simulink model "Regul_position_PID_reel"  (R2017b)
settings: Solver=ode5  StartTime=0.0  StopTime=inf  FixedStep=0.005  RelTol=1e-3  AbsTol=1e-6
undefined symbols (not defined in the file or in its folder): RTDAC4PCIBaseAddress

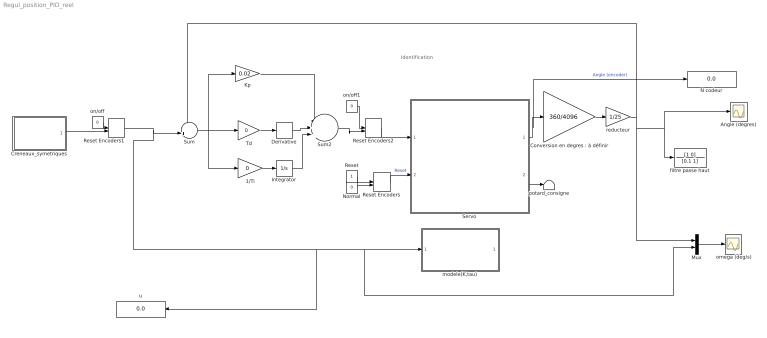
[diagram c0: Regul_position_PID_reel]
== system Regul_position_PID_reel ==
  note: Identification
  " omega (deg/s)" : Scope
  1/Ti : Gain  Gain=0
  Angle (degres) : Scope
  "Conversion en degres : à définir" : Gain  Gain=360/4096
  Creneaux_symetriques : Subsystem
  Derivative : Derivative
  Integrator : Integrator
  Kp : Gain  Gain=0.02
  Mux : Mux  Inputs=2
  N codeur : Display
  Normal : Constant  Value=0
  Reset : Constant
  Reset Encoders : ManualSwitch  CurrentSetting=0
  Reset Encoders1 : ManualSwitch  CurrentSetting=0
  Reset Encoders2 : ManualSwitch  CurrentSetting=0
  Servo : Subsystem  mask{BaseAddress=RTDAC4PCIBaseAddress(-1,-1), T0=0.005}
      mask prompts: BaseAddress "Base Address:"; T0 "Sampling Period:"
  Sum : Sum  Inputs=-+|
  Sum2 : Sum  Inputs=|+||+|+||
  Td : Gain  Gain=0
  filtre passe haut : TransferFcn  Numerator=[1 0]  Denominator=[0.1 1]
  modele(K,tau) : Subsystem
  on/off : Constant  Value=0
  on/off1 : Constant  Value=0
  potard_consigne : Terminator
  reducteur : Gain  Gain=1/25
  u : Display
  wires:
  Reset Encoders/1 -> Servo/2(Reset Encoder)  "Reset"
  Normal/1 -> Reset Encoders/2
  Reset/1 -> Reset Encoders/1
  Servo/2(Set-up) -> potard_consigne/1
  Servo/1(Codeur_angulaire) -> N codeur/1, "Conversion en degres : à définir"/1  "Angle (encoder)"
  "Conversion en degres : à définir"/1 -> reducteur/1
  Mux/1 -> " omega (deg/s)"/1
  on/off/1 -> Reset Encoders1/1
  Creneaux_symetriques/1(u) -> Reset Encoders1/2
  Reset Encoders1/1 -> Sum/2, Mux/2, modele(K,tau)/1(u), u/1
  Td/1 -> Derivative/1
  Integrator/1 -> Sum2/3
  Derivative/1 -> Sum2/2
  Kp/1 -> Sum2/1
  1/Ti/1 -> Integrator/1
  Sum/1 -> 1/Ti/1, Kp/1, Td/1
  reducteur/1 -> Mux/1, Angle (degres)/1, filtre passe haut/1, Sum/1
  Sum2/1 -> Reset Encoders2/2
  Reset Encoders2/1 -> Servo/1(PWM Control)
  on/off1/1 -> Reset Encoders2/1

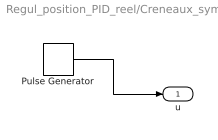
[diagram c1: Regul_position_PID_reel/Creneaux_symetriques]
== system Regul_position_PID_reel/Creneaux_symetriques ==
  Pulse Generator : DiscretePulseGenerator  PulseType=Time based  Amplitude=20  Period=0.005*floor(15/0.005)  PulseWidth=50  PhaseDelay=0.005*floor(0*15/0.005/4)
  u : Outport
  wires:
  Pulse Generator/1 -> u/1

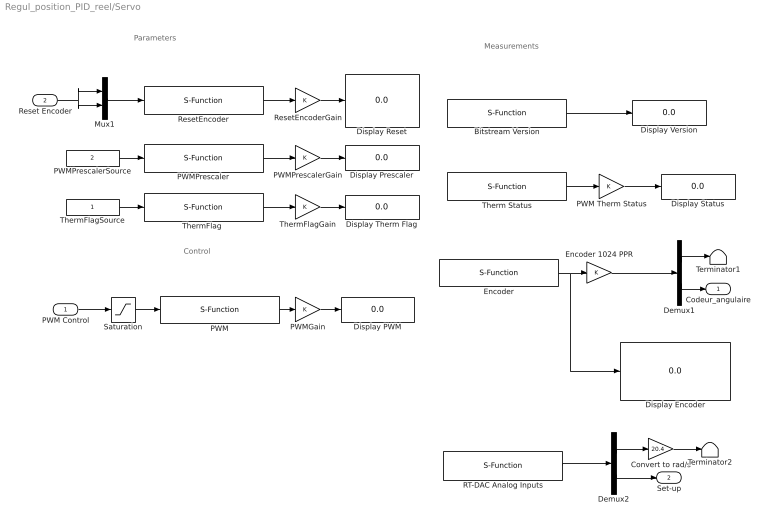
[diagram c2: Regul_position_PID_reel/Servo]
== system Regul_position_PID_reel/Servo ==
  note: Parameters
  note: Control
  note: Measurements
  PWM Control : Inport
  Reset Encoder : Inport  Port=2
  Bitstream Version : S-Function  FunctionName=Servo_BitstreamVersion  Parameters=BaseAddress, T0  SFunctionDeploymentMode=off  EnableBusSupport=off
  Convert to rad/s : Gain  Gain=20.4
  Demux1 : Demux  Outputs=2
  Demux2 : Demux  Outputs=2
  Display Encoder : Display
  Display PWM : Display
  Display Prescaler : Display
  Display Reset : Display
  Display Status : Display
  Display Therm Flag : Display
  Display Version : Display
  Encoder : S-Function  FunctionName=Servo_Encoder  Parameters=BaseAddress, T0  SFunctionDeploymentMode=off  EnableBusSupport=off
  Encoder 1024 PPR : Gain
  Mux1 : Mux  Inputs=2
  PWM : S-Function  FunctionName=Servo_PWM  Parameters=BaseAddress, T0  SFunctionDeploymentMode=off  EnableBusSupport=off
  PWM Therm Status : Gain
  PWMGain : Gain
  PWMPrescaler : S-Function  FunctionName=Servo_PWMPrescaler  Parameters=BaseAddress, T0  SFunctionDeploymentMode=off  EnableBusSupport=off
  PWMPrescalerGain : Gain
  PWMPrescalerSource : Constant  Value=2
  RT-DAC Analog Inputs : S-Function  FunctionName=servo_analoginputs  Parameters=BaseAddress, [1 0], [1 1], T0  SFunctionDeploymentMode=off  EnableBusSupport=off
  ResetEncoder : S-Function  FunctionName=Servo_ResetEncoder  Parameters=BaseAddress, T0  SFunctionDeploymentMode=off  EnableBusSupport=off
  ResetEncoderGain : Gain
  Saturation : Saturate  UpperLimit=1  LowerLimit=-1
  Terminator1 : Terminator
  Terminator2 : Terminator
  Therm Status : S-Function  FunctionName=Servo_PWMTherm  Parameters=BaseAddress, T0  SFunctionDeploymentMode=off  EnableBusSupport=off
  "ThermFlag " : S-Function  FunctionName=Servo_ThermFlag  Parameters=BaseAddress, T0  SFunctionDeploymentMode=off  EnableBusSupport=off
  ThermFlagGain : Gain
  ThermFlagSource : Constant
  Codeur_angulaire : Outport
  Set-up : Outport  Port=2
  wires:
  Encoder/1 -> Encoder 1024 PPR/1, Display Encoder/1
  Saturation/1 -> PWM/1
  PWM/1 -> PWMGain/1
  PWMGain/1 -> Display PWM/1
  ResetEncoder/1 -> ResetEncoderGain/1
  PWMPrescaler/1 -> PWMPrescalerGain/1
  Mux1/1 -> ResetEncoder/1
  PWMPrescalerSource/1 -> PWMPrescaler/1
  ResetEncoderGain/1 -> Display Reset/1
  PWMPrescalerGain/1 -> Display Prescaler/1
  PWM Control/1 -> Saturation/1
  Encoder 1024 PPR/1 -> Demux1/1
  Therm Status/1 -> PWM Therm Status/1
  PWM Therm Status/1 -> Display Status/1
  Bitstream Version/1 -> Display Version/1
  Reset Encoder/1 -> Mux1/1, Mux1/2
  "ThermFlag "/1 -> ThermFlagGain/1
  ThermFlagSource/1 -> "ThermFlag "/1
  ThermFlagGain/1 -> Display Therm Flag/1
  Demux1/1 -> Terminator1/1
  Demux1/2 -> Codeur_angulaire/1
  RT-DAC Analog Inputs/1 -> Demux2/1
  Demux2/2 -> Set-up/1
  Demux2/1 -> Convert to rad/s/1
  Convert to rad/s/1 -> Terminator2/1

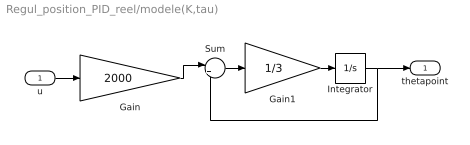
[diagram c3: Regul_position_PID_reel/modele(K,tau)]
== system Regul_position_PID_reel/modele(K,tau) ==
  u : Inport
  Gain : Gain  Gain=2000
  Gain1 : Gain  Gain=1/3
  Integrator : Integrator
  Sum : Sum  Inputs=|+-
  thetapoint : Outport
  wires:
  Gain/1 -> Sum/1
  Gain1/1 -> Integrator/1
  Integrator/1 -> thetapoint/1, Sum/2
  Sum/1 -> Gain1/1
  u/1 -> Gain/1
